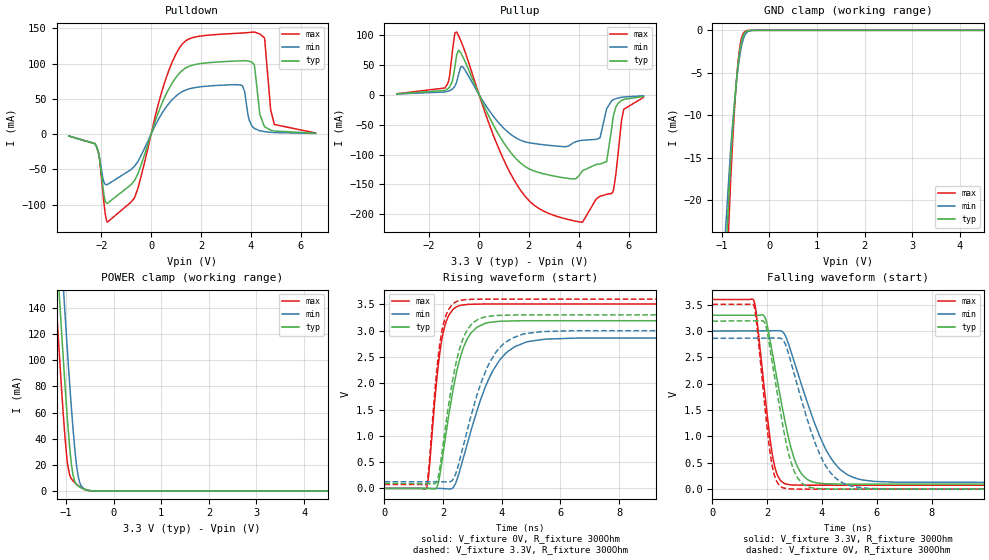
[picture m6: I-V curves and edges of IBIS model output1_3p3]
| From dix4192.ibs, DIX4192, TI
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|   output1_3p3 Model
[Model]   output1_3p3
Model_type   3-state
Polarity   Non-Inverting
Vmeas = 1.65
Vref = 0
Cref = 2pF
Rref = 100000
|   typ   min   max
C_comp   31.0199pF   25.0988pF   36.7824pF
|C_comp_pullup   31.4507pF   25.5641pF   37.4659pF
|C_comp_pulldown   31.7373pF   25.9207pF   37.466pF
| Where nom  PVT is Nominal Process, 3.3V, 27C
|   Fast PVT is Strong Process,  3.6V, -40C
|   Slow PVT is Weak Process,   3.0V, 105C
[Voltage Range]   3.3   3   3.6
[Temperature Range]   27   105   -40
[Pullup Reference]   3.3   3   3.6
[Pulldown Reference]   0   -0   0
[Power Clamp Reference]   3.3   3   3.6
[GND Clamp Reference]   0   0   0
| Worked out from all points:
|   slope of the pulldown table from 0 to 0.495 V, typ, clamps not added: 10.2 ohm
|   slope of the pullup table from 0 to 0.495 V, typ, clamps not added: 11.2 ohm
|   GND clamp passes 1 mA (typ) near -0.57 V on its own axis
|   POWER clamp passes 1 mA (typ) near -0.59 V on its own axis
|   falling waveform, V_fixture 3.3V, R_fixture 300Ohm: 20-80 % time 733ps typ, 1.21ns min, 458ps max; typ from 3.3 V to 0.095 V
|   rising waveform, V_fixture 0V, R_fixture 300Ohm: 20-80 % time 625ps typ, 1.07ns min, 374ps max; typ from 0 V to 3.19 V
|   rising waveform, V_fixture 3.3V, R_fixture 300Ohm: 20-80 % time 590ps typ, 980ps min, 360ps max; typ from 0.095 V to 3.3 V
|   falling waveform, V_fixture 0V, R_fixture 300Ohm: 20-80 % time 664ps typ, 1.07ns min, 422ps max; typ from 3.19 V to 0 V
[Pulldown]
|   Voltage   I(typ)   I(min)   I(max)
-3.3V     -2.85mA    -2.595mA   -2.851mA
-2.191V   -18.04mA   -17.58mA   -17.54mA
-1.756V   -98.15mA   -71.47mA   -124.9mA
-656.7mV  -65.34mA   -45.09mA   -89.63mA
432.3mV   43.23mA    29.27mA    60.55mA
1.214V    89.07mA    59.43mA    126mA
3.64V     104mA      68.94mA    143.3mA
4.125V    99.15mA    8.551mA    144.6mA
4.551V    10.64mA    3.483mA    135.2mA
4.798V    5.618mA    2.568mA    34.1mA
4.947V    4.357mA    2.216mA    13.59mA
6.6V      1.224mA    869.1uA    1.663mA
[GND Clamp]
|   Voltage   I(typ)   I(min)   I(max)
-3.3V     -1.043A    -967.2mA   -1.114A
-1.152V   -52.29mA   -43.66mA   -63.35mA
-815.1mV  -15.23mA   -13.91mA   -17.52mA
-765.6mV  -11mA      -10.44mA   -12.23mA
-726mV    -8.002mA   -7.941mA   -8.52mA
-686.4mV  -5.423mA   -5.733mA   -5.395mA
-656.7mV  -3.815mA   -4.304mA   -3.522mA
-627mV    -2.518mA   -3.091mA   -2.102mA
-587.4mV  -1.291mA   -1.835mA   -903.6uA
-498.3mV  -177.8uA   -394.8uA   -74.75uA
-260.7mV  0A         -937.5nA   0A
6.6V      0A         0A         0A
[Pullup]
|   Voltage   I(typ)   I(min)   I(max)
-3.3V     1.193mA    955.2uA    1.362mA
-1.369V   6.903mA    4.325mA    11mA
-1.073V   21.93mA    9.068mA    70.24mA
-894.3mV  66.92mA    21.2mA     104.3mA
-646.8mV  62.78mA    45.89mA    81.1mA
1.601V    -111.6mA   -74.87mA   -155.5mA
4.135V    -128.1mA   -76.3mA    -212.9mA
4.848V    -115.8mA   -72.43mA   -169.9mA
5.115V    -112mA     -24.67mA   -166.5mA
5.362V    -43.67mA   -9.248mA   -163mA
5.808V    -8.044mA   -4.049mA   -24.46mA
6.6V      -3.081mA   -1.983mA   -4.664mA
[POWER Clamp]
|   Voltage   I(typ)   I(min)   I(max)
-3.3V     1.547A     1.6A       1.506A
-1.261V   221.8mA    278.9mA    176.5mA
-1.201V   185.4mA    242.4mA    140.3mA
-1.181V   173.4mA    230.3mA    128.4mA
-1.092V   120.7mA    176.8mA    76.94mA
-1.063V   103.7mA    159.3mA    60.97mA
-1.033V   87.14mA    142.1mA    46.08mA
-963.6mV  51.24mA    103.1mA    19.41mA
-854.7mV  12.41mA    48.08mA    7.805mA
-745.8mV  3.823mA    11.52mA    4.15mA
-607.2mV  1.171mA    1.445mA    1.051mA
6.6V      0A         0A         0A
[Ramp]
R_load = 300
|   typ   min   max
dV/dt_r   1.91352/6.24592e-10   1.71722/1.06485e-09   2.10458/3.74149e-10
dV/dt_f   1.92296/7.31318e-10   1.72388/1.21296e-09   2.11532/4.57712e-10
[Falling Waveform]
V_fixture = 3.3V
V_fixture_min = 3V
V_fixture_max = 3.6V
R_fixture = 300Ohm
C_fixture = 0F
|   Time   V(typ)   V(min)   V(max)
0s        3.3V       3V         3.6V
1.513ns   3.3V       3.003V     3.578V
1.916ns   3.263V     3.004V     1.811V
2.181ns   2.61V      3.005V     684.3mV
2.635ns   1.33V      2.938V     106mV
2.994ns   571.8mV    2.406V     79.12mV
3.416ns   204.4mV    1.726V     75.31mV
4.222ns   102.5mV    676.1mV    75.26mV
5.119ns   96.17mV    228.2mV    75.21mV
17.86ns   95.07mV    126.9mV    74.47mV
[Rising Waveform]
V_fixture = 0V
V_fixture_min = 0V
V_fixture_max = 0V
R_fixture = 300Ohm
C_fixture = 0F
|   Time   V(typ)   V(min)   V(max)
0s        -613.6nV   -161.6nV   -22.6nV
1.44ns    265.1uV    146uV      12.88mV
1.785ns   15.18mV    181uV      2.072V
1.955ns   494.5mV    -1.419mV   2.819V
2.181ns   1.344V     -9.656mV   3.276V
2.53ns    2.376V     263mV      3.47V
2.965ns   2.961V     1.123V     3.501V
3.656ns   3.16V      2.194V     3.506V
4.823ns   3.187V     2.779V     3.507V
17.86ns   3.189V     2.862V     3.508V
[Rising Waveform]
V_fixture = 3.3V
V_fixture_min = 3V
V_fixture_max = 3.6V
R_fixture = 300Ohm
C_fixture = 0F
|   Time   V(typ)   V(min)   V(max)
0s        95.07mV    126.9mV    74.47mV
1.43ns    89.24mV    125.4mV    82.4mV
1.513ns   88.9mV     125.3mV    387.2mV
1.769ns   110.7mV    125mV      2.159V
1.94ns    595.4mV    124.8mV    2.932V
2.497ns   2.519V     395.1mV    3.562V
2.904ns   3.076V     1.278V     3.593V
3.518ns   3.269V     2.315V     3.599V
4.677ns   3.298V     2.925V     3.599V
17.86ns   3.3V       3V         3.6V
[Falling Waveform]
|Gnd
V_fixture = 0V
V_fixture_min = 0V
V_fixture_max = 0V
R_fixture = 300Ohm
C_fixture = 0F
|   Time   V(typ)   V(min)   V(max)
0s        3.189V     2.862V     3.508V
1.513ns   3.194V     2.865V     3.484V
1.903ns   3.161V     2.866V     1.637V
2.14ns    2.55V      2.866V     575.6mV
2.565ns   1.226V     2.842V     29.35mV
2.872ns   509.8mV    2.4V       4.766mV
3.242ns   128.2mV    1.715V     874.3uV
4.103ns   6.463mV    472.1mV    822.8uV
5.02ns    1.257mV    66.39mV    767.9uV
17.86ns   -180.4nV   -90.69nV   -23.18nV
